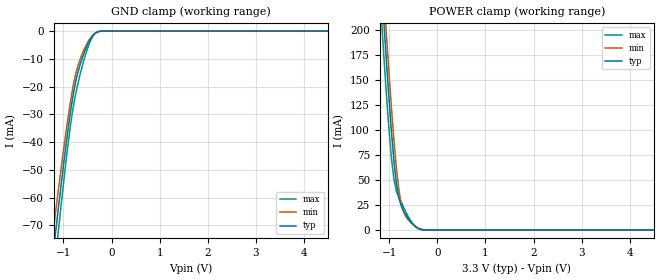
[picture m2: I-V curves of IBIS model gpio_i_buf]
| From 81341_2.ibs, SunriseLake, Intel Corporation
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[Model]   gpio_i_buf
Model_type   Input
Vinl = 1.155V
Vinh = 1.650V
|Vmeas = 1.320V
|Vref = 0.000V
|Cref = 10.000pF
|Rref = 50.000Ohm
|   typ   min   max
C_comp   5.000pF   4.750pF   5.250pF
[Voltage Range]   3.300V   3.000V   3.600V
[Temperature Range]   60.0   110.0   -5.0
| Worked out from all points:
|   GND clamp passes 1 mA (typ) near -0.35 V on its own axis
|   POWER clamp passes 1 mA (typ) near -0.36 V on its own axis
[GND Clamp]
|   Voltage   I(typ)   I(min)   I(max)
-3.3V     -392.6mA   -362.9mA   -431.7mA
-1.25V    -85.75mA   -77.5mA    -96.38mA
-1.2V     -78.06mA   -70.39mA   -87.87mA
-1.15V    -70.46mA   -63.37mA   -79.46mA
-1.1V     -62.97mA   -56.47mA   -71.17mA
-900mV    -34.89mA   -30.68mA   -40.16mA
-750mV    -18.5mA    -15.77mA   -23mA
-650mV    -11.89mA   -9.961mA   -15.39mA
-500mV    -4.899mA   -4.134mA   -6.303mA
-400mV    -1.867mA   -1.637mA   -2.26mA
-300mV    -357.3uA   -362.2uA   -330uA
6.6V      0A         0A         0A
[POWER Clamp]
|   Voltage   I(typ)   I(min)   I(max)
-3.3V     1.906A     1.939A     1.845A
-1.15V    237.5mA    264.5mA    202.2mA
-1.1V     199.5mA    226.3mA    164.9mA
-1.05V    162.8mA    189.2mA    129.5mA
-950mV    95.69mA    119.4mA    69.99mA
-900mV    67.74mA    88.25mA    50.02mA
-850mV    45.99mA    61.3mA     38.57mA
-800mV    32.08mA    40.38mA    32.57mA
-750mV    24.08mA    25.9mA     27.87mA
-700mV    18.75mA    17.74mA    22.46mA
-400mV    1.715mA    1.884mA    1.374mA
6.6V      0A         0A         0A
